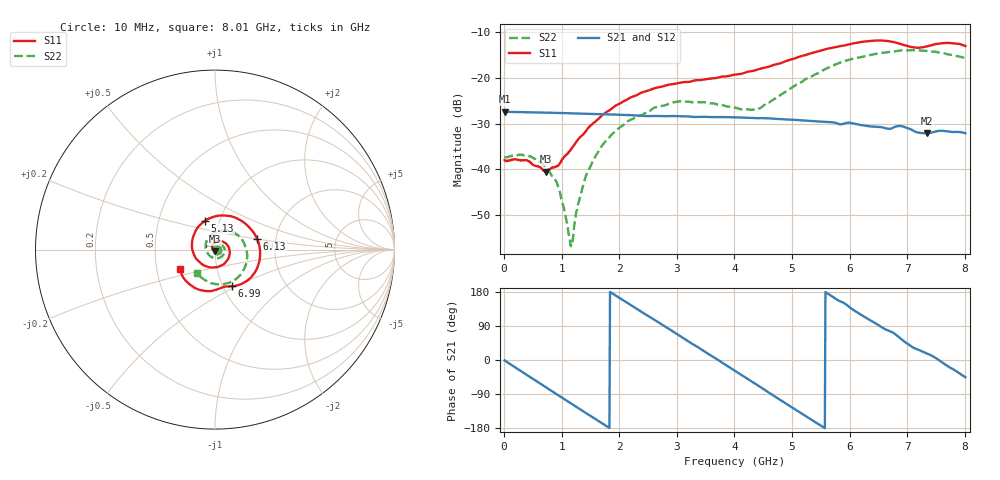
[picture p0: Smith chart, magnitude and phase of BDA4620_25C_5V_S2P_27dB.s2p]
!Agilent Technologies,E5071B,MY42404982,A.09.10
!Date: Wed May 06 09:04:20 2026
!Data & Calibration Information:
!Freq	S11:SOLT2(ON)	S21:SOLT2(ON)	S12:SOLT2(ON)	S22:SOLT2(ON)
# Hz S RI R 50
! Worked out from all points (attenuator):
!   801 points, 10 MHz to 8.01 GHz, reference 50 ohm
!   highest |S21| = -27.39 dB at 10 MHz (marker M1); lowest = -32.1 dB at 7.34 GHz (marker M2)
!   lowest |S11| = -40.5 dB at 720 MHz (marker M3), VSWR 1.02, Z = 49.8 - j0.934 ohm
!   |S11| at or under -10 dB: start of sweep to end of sweep
!   |S22| runs from -56.8 to -13.9 dB; largest |S21 - S12| = 0.00021
!   S11 on the Smith chart (normalised r, x): 10 MHz: 1.03, -0.00; 5.13 GHz: 0.85, +0.28; 6.13 GHz: 1.60, +0.20; 6.99 GHz: 1.10, -0.47; 8.01 GHz: 0.66, -0.15
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1e7  0.0126 -0.000784  0.0427 -0.000868  0.0428 -0.000905  0.0135 -0.000464
4.3e8  0.00855 -0.00891  0.0309 -0.0286  0.0309 -0.0287  0.0132 -0.00472
7.2e8  -0.00153 -0.00937  0.0134 -0.0395  0.0134 -0.0396  0.0084 -0.00684
9.4e8  -0.00994 -0.00469  -0.00209 -0.0413  -0.0021 -0.0414  0.00332 -0.00549
1.16e9  -0.0156 0.00551  -0.0169 -0.0374  -0.017 -0.0374  -0.00123 -0.000765
1.19e9  -0.016 0.00724  -0.0188 -0.0364  -0.0189 -0.0365  -0.00167 7.12e-05
1.35e9  -0.0164 0.0169  -0.0277 -0.0298  -0.0278 -0.0298  -0.00323 0.00487
1.54e9  -0.0117 0.0294  -0.0354 -0.0194  -0.0355 -0.0194  -0.00297 0.0119
1.77e9  0.00132 0.042  -0.0397 -0.00452  -0.0398 -0.00453  0.00113 0.0205
2.14e9  0.0349 0.0469  -0.0343 0.0193  -0.0343 0.0193  0.0169 0.0288
2.68e9  0.0788 0.00728  -0.00628 0.0378  -0.00625 0.0378  0.0442 0.0192
3.08e9  0.0751 -0.0482  0.0185 0.0333  0.0186 0.0333  0.0549 -0.00756
4.01e9  -0.0692 -0.0837  0.0325 -0.0178  0.0326 -0.0179  -0.0105 -0.0463
4.43e9  -0.1249 -0.00615  0.0128 -0.0339  0.0128 -0.034  -0.0448 -0.0115
5.13e9  -0.0549 0.1614  -0.0255 -0.0233  -0.0256 -0.0233  -0.014 0.087
5.35e9  0.01 0.1874  -0.0315 -0.0121  -0.0315 -0.0121  0.0233 0.102
6.13e9  0.2355 0.0584  -0.0182 0.0252  -0.0182 0.0254  0.1622 0.0353
6.68e9  0.1939 -0.161  0.00628 0.027  0.00629 0.0271  0.1694 -0.0894
6.99e9  0.0927 -0.2042  0.0204 0.0198  0.0205 0.02  0.1265 -0.1563
7.34e9  0.0164 -0.2205  0.0237 0.00734  0.0237 0.00745  0.0442 -0.1929
7.66e9  -0.0984 -0.2201  0.0257 -0.00543  0.0258 -0.00543  -0.0348 -0.1813
8.01e9  -0.194 -0.1108  0.0174 -0.0177  0.0175 -0.0178  -0.1027 -0.1283
